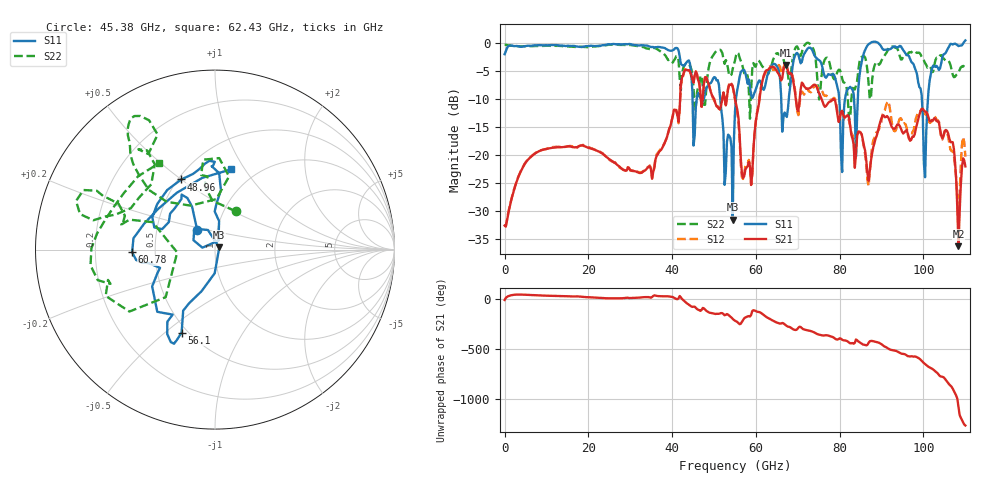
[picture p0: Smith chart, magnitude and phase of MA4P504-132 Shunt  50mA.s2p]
!Keysight Technologies,N5247B,US61255204,A.15.70.20
!Date: Friday, October 21, 2022 14:59:22
!Correction: S11(C  4-Port  )
!S31(C  4-Port  )
!S13(C  4-Port  )
!S33(C  4-Port  )
!S2P File: Measurements: S11, S31, S13, S33:
# Hz S  dB  R 50
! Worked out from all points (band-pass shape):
!   401 points, 10 MHz to 110 GHz, reference 50 ohm
!   highest |S21| = -3.95 dB at 67.1 GHz (marker M1); lowest = -36.2 dB at 108.4 GHz (marker M2)
!   |S21| within 3 dB of the highest: 42.14 GHz to 45.04 GHz (2.903 GHz wide, 6.66 % of centre); 61.51 GHz to 68.93 GHz (7.422 GHz wide, 11.4 % of centre)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
!   lowest |S11| = -31.5 dB at 54.46 GHz (marker M3), VSWR 1.05, Z = 52.4 + j1.24 ohm
!   |S11| at or under -10 dB: 51.49 GHz to 55.24 GHz (3.757 GHz wide, 7.04 % of centre); 66.03 GHz to 67.85 GHz (1.816 GHz wide, 2.71 % of centre); 79.87 GHz to 81.28 GHz (1.404 GHz wide, 1.74 % of centre)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
!   |S22| runs from -13.6 to 0.0 dB; largest |S21 - S12| = 0.24
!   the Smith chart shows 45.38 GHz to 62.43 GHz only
!   S11 on the Smith chart (normalised r, x): 45.38 GHz: 0.80, +0.18; 48.96 GHz: 0.52, +0.50; 56.1 GHz: 0.46, -0.57; 60.78 GHz: 0.37, -0.01; 62.43 GHz: 0.77, +0.87
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1e7  -2.02 -179.9  -32.55 -5.1  -32.52 -5.0  -0.33 179.9
1.843332e10  -0.73 118.0  -18.26 27.2  -18.29 27.3  -0.71 124.6
3.685665e10  -0.74 115.5  -19.45 32.9  -19.29 32.9  -1.32 122.3
4.373102e10  -3.24 17.5  -4.90 -44.8  -4.74 -42.7  -4.02 81.7
4.538088e10  -16.53 131.9  -5.81 -72.8  -5.72 -72.0  -12.29 61.8
4.895555e10  -7.26 115.6  -8.01 -133.4  -7.95 -131.6  -3.64 133.8
5.445505e10  -31.48 26.3  -7.73 164.7  -7.81 164.0  -4.61 160.7
5.5005e10  -12.26 -107.9  -9.92 146.6  -10.16 144.8  -3.13 166.5
5.61049e10  -6.05 -111.9  -16.36 111.3  -17.26 114.9  -2.66 153.5
6.077948e10  -6.70 -178.1  -10.55 -126.9  -10.12 -122.3  -3.24 179.4
6.242932e10  -6.84 78.9  -4.90 -174.6  -5.15 -168.2  -4.83 122.8
6.462912e10  -3.83 16.5  -4.58 134.0  -4.72 155.4  -2.10 62.8
6.71039e10  -12.73 -40.5  -3.95 101.7  -3.63 102.2  -4.29 45.6
7.342832e10  -1.27 138.9  -7.71 37.8  -8.41 36.1  -0.67 108.7
8.112762e10  -10.72 -28.7  -13.32 -51.6  -13.64 -52.2  -7.10 -125.4
8.525225e10  -3.36 39.3  -16.28 -85.9  -16.38 -84.5  -2.50 -23.0
9.185165e10  -1.16 91.0  -13.76 -140.3  -11.11 -134.2  -0.76 83.9
9.872602e10  -6.98 150.1  -13.64 132.6  -12.44 132.0  -1.73 176.9
1.003759e11  -23.94 -16.4  -12.23 70.9  -12.69 72.9  -3.59 -156.2
1.036756e11  -4.82 -33.8  -14.19 -38.7  -14.05 -35.4  -2.59 -89.7
1.083502e11  -0.56 22.2  -36.23 -1.3  -34.02 4.8  -5.18 -5.4
1.1e11  0.43 54.4  -22.02 172.9  -20.27 175.4  -4.08 16.4
